(* Logix 5000 AddOnInstructionDefinition export EH_PicomagInsertion_DMI_IOL; software revision 38.00 *)

TYPE EH_CommAOI_Data :
STRUCT
   Device_Comm_Error : BOOL;
   CommSuccess : BOOL;
   CommFailed : BOOL;
   CommTimeOut : BOOL;
   StateDone : BOOL;
   NewState : BOOL;
   OldState : SINT;
   PortSize : SINT;
   DevicePort : SINT;
   MaxState : SINT;
   State : SINT;
   VendorID : INT;
   DeviceID : DINT;
   CyclicData : INT[16];
   AcyclicData : DINT[8];
   ReplayIndex : INT;
   AOI_Diagnostic : DINT;
   ConnectionStatus : DINT;
   OutputData : INT[16];
END_STRUCT
END_TYPE

ADD_ON_INSTRUCTION EH_PicomagInsertion_DMI_IOL   (* revision 1.0, vendor Endress+Hauser *)
// Picomag Insertion DMI Rev 1 IO-Link
VAR_IN_OUT
   DataToSend : INT[10]; {required}
   CommAOIBusy : DINT; {required}
   ActiveComPort : DINT; {required}
   DeviceAOISendRequest : DINT; {required}
   CommError : INT; {required}
   DeviceData : EH_CommAOI_Data; {required}
END_VAR
VAR_INPUT
   iSetSimulation : BOOL; {visible}
   iSimulation_OnOff : SINT; {access None, visible}
   iSimulationValue_FlowVelocity : REAL; {visible}
   iSimulationValue_Temperature : REAL; {visible}
   iSimulationValue_Conductivity : REAL; {visible}
   iSetTotalizerPresetValue : BOOL; {visible}
   iTotalizerPresetValue : REAL; {visible}
   iResetTotalizer : BOOL; {visible}
   iReadExtendedProcessData : BOOL; {access None, visible}
   iSetUnits : BOOL; {visible}
   iUnitConductivity : SINT; {visible}
   iUnitTotalizer : INT; {access None, visible}
   iUnitTemperature : SINT; {visible}
   iUnitFlowVelocity : INT; {visible}
   iUnitVolumeFlow : SINT; {visible}
END_VAR
VAR_OUTPUT
   qVendor_ID : DINT; {access Read Only, visible}
   qDevice_ID : DINT; {access Read Only, visible}
   qConductivity : REAL; {access None, visible}
   qVolumeTotalizer : REAL; {access None, visible}
   qTemperature : REAL; {visible}
   qFlowVelocity : REAL; {visible}
   qExtendedDeviceStatus : INT; {access Read Only, visible}
   qRelativeFlowRate : REAL; {access None, visible}
   qVolumeFlow : REAL; {access None, visible}
   qUnitConductivity : SINT; {access None, visible}
   qUnitTotalizer : INT; {access None, visible}
   qUnitTemperature : SINT; {access None, visible}
   qUnitFlowVelocity : INT; {access None, visible}
   qUnitVolumeFlow : SINT; {access None, visible}
   qAOI_Diagnostic : DINT; {access Read Only, visible}
END_VAR
VAR_IN_OUT
   qAOI_Diagnostic_String : STRING; {required}
END_VAR
VAR_OUTPUT
   qActual_Diagnostics_Code : DINT; {access Read Only, visible}
END_VAR
VAR_IN_OUT
   qActual_Diagnostics_String : STRING; {required}
END_VAR
VAR_OUTPUT
   qCommError : DINT; {access None}
   qCommunicationBusy : DINT; {access Read Only, visible}
   qDeviceConnectionError : BOOL; {access Read Only, visible}
END_VAR
VAR
   Temp_DINT : DINT; {access None}
   CMD_Index : INT; {access None}
   CMD_Subindex : INT; {access None}
   CMD_ByteLength : INT; {access None}
   oldCondStatus : INT; {access None}
   SetSimulation : SINT; {access None}
   SetTotalizerPresetValue : SINT; {access None}
   oldSetTotalizerPresetValue : SINT; {access None}
   oldSetSimulation : SINT; {access None}
   Trigger : BOOL; {access None}
   CMD_Rd : BOOL; {access None}
   CMD_Wr : BOOL; {access None}
   SimulationDINT : DINT; {access None}
   AOI_Prio : BOOL; {access None}
   StateMin : DINT; {access None}
   firstTimeDone : BOOL; {access None}
   CondStatusChanged : BOOL; {access None}
   Calc_Temperature : DINT; {access None}
   Calc_ExtendedDeviceStatus : DINT; {access None}
   CondStatusActive : BOOL; {access None}
   ActiveAOI : BOOL; {access None}
   TotActive : BOOL; {access None}
   Skip : BOOL; {access None}
   SetPulseSimulation : SINT; {access None}
   Calc_FlowVelocity : SINT; {access None}
   Calc_Totalizer : SINT; {access None}
   Calc_Conductivity : SINT; {access None}
   TotPresetChanged : BOOL; {access None}
   DeviceID : DINT; {access None}
   ResetTotalizerValue : SINT; {access None}
   oldResetTotalizerValue : SINT; {access None}
   SetUnits : SINT; {access None}
   oldSetUnits : SINT; {access None}
   SimChanged : BOOL; {access None}
   TRUE : BOOL := 1; {access None}
   FALSE : BOOL; {access None}
   SimActive : BOOL; {access None}
   temp_string1 : STRING; {access None}
   temp_string2 : STRING; {access None}
   tGradientConductivity : REAL; {access None}
   qConductivityTemp : REAL; {access None}
   qTemperatureTemp : REAL; {access None}
   qFlowVelocityTemp : REAL; {access None}
   tGradientFlowVelocity : REAL; {access None}
   qTotalizerTemp : REAL; {access None}
   qVolumeFlowTemp : REAL; {access None}
   qRelativeFlowRateTemp : REAL; {access None}
   ReadExtendedProcessData : SINT; {access None}
   oldReadExtendedProcessData : SINT; {access None}
   SetSimulation_OnOff : SINT; {access None}
   TotResetChanged : BOOL; {access None}
   UnitChanged : BOOL; {access None}
   UnitActive : BOOL; {access None}
   TotPresetActive : BOOL; {access None}
   TotResetActive : BOOL; {access None}
   ReadProcessDataChanged : BOOL; {access None}
   ReadProcessDataActive : BOOL; {access None}
   iSimulationValue_FlowVelocityTemp : REAL; {access None}
   SimulationValue_ConductivityTemp : REAL; {access None}
   qRelativeFlowRate_DINT : DINT; {access None}
   qVolumeFlow_DINT : DINT; {access None}
   iTotalizerPresetValueTemp : REAL; {access None}
   unit_check : BOOL; {access None}
   init_qUnits : BOOL; {access None}
   Underline_string : STRING; {access None}
END_VAR

ROUTINE Logic   (* structured text *)
// Picomag Communication via AL1323
   // =======================================================================
   // Endress+Hauser Digital Solutions
   // ©Copyright (2024) All Rights Reserved
   // =======================================================================
   // Name:                EH_PicomagInsertion_DMI_IOL
   // Version:             1.0
   // Datum:               11.2025
   // Library:             01.01.00
   // Engineering:         Studio5000 V38.00.00
   // Author:              EH
   // =======================================================================
   
   qAOI_Diagnostic := DeviceData.AOI_Diagnostic;
   qCommunicationBusy := CommAOIBusy;
   DeviceID := 9728001;
   StateMin := 0;
   DeviceData.MaxState := 98;
   temp_string1 := 'Error in step ';
   Underline_string := '----';
   
   if DeviceData.DevicePort = 0 or DeviceData.DeviceID <> DeviceID or DeviceData.ConnectionStatus <> 1 then
   
   	qVendor_ID := DeviceData.VendorID;
   	qDevice_ID := DeviceData.DeviceID;
   	qFlowVelocity := 0;
   	qTemperature := 0;
   	qFlowVelocity := 0;
   	qVolumeTotalizer := 0;
   	qRelativeFlowRate := 0;
   	qVolumeFlow := 0;
   	qConductivity := 0;
   	qUnitConductivity := 0;
   	qUnitTotalizer := 0;
   	qUnitTemperature := 0;
   	qUnitFlowVelocity := 0;
   	qUnitVolumeFlow := 0;
   	qExtendedDeviceStatus := 0;
   	qActual_Diagnostics_Code	:= 0;
   	DELETE(qActual_Diagnostics_String,1,1,qActual_Diagnostics_String);
   	oldCondStatus := 0;
   	CondStatusChanged := FALSE;
   	init_qUnits := FALSE;
   
   	if DeviceData.DevicePort = 0 then
   
   		qAOI_Diagnostic_String := 'Device port is zero';
   
   	elsif DeviceData.ConnectionStatus <> 1 then
   
   		qAOI_Diagnostic_String := 'No device connected';
   
   	elsif DeviceData.DeviceID <> DeviceID then
   
   		qAOI_Diagnostic_String := 'Wrong device ID';
   
   	end_if;
   
   else
   
   	if qActual_Diagnostics_Code = 0  then
   
   		CONCAT(Underline_string,Underline_string,qActual_Diagnostics_String);
   
   	end_if;
   
   	DELETE(qAOI_Diagnostic_String,1,1,qAOI_Diagnostic_String);
   	DeviceData.AOI_Diagnostic.1 := FALSE;
   	qDeviceConnectionError := FALSE;
   	DeviceData.AOI_Diagnostic.2  := FALSE;
   
   end_if;
   
   // Case device disconnected during communication to avoid blocking the communication
   if (DeviceData.AOI_Diagnostic.0 or qDeviceConnectionError or DeviceData.AOI_Diagnostic.2) and ActiveAOI and ActiveComPort = DeviceData.DevicePort and CommAOIBusy = 1 then
   
   	DeviceData.State := 0;
   	CommAOIBusy := 0;
   	DeviceAOISendRequest.[DeviceData.DevicePort] := 0;
   	ActiveComPort := 0;
   	ActiveAOI := 0;
   	DataToSend[0] := 0;
   	DataToSend[1] := 0;
   	DataToSend[2] := 0;
   	DataToSend[3] := 0;
   	DataToSend[4] := 0;
   	DataToSend[5] := 0;
   	DataToSend[6] := 0;
   	DataToSend[7] := 0;
   	DataToSend[8] := 0;
   	DataToSend[9] := 0;
   	DeviceData.StateDone := FALSE;
   	DeviceData.NewState := FALSE;
   	DeviceData.OldState := 0;
   	ActiveAOI := FALSE;
   
   end_if;
   
   if not DeviceData.AOI_Diagnostic.0
   	and not qDeviceConnectionError
   	and not DeviceData.AOI_Diagnostic.2
   	and DeviceData.DevicePort > 0 then
   
   	//*********************************
   	//Vendor ID
   	//*********************************
   
   		qVendor_ID := DeviceData.VendorID;
   
   	//*********************************
   	//Device ID
   	//*********************************
   
   		qDevice_ID := DeviceData.DeviceID;
   
   	//*********************************
   	// Picomag Insertion
   	//*********************************
   		Calc_Conductivity		    := 0;
   		Calc_Totalizer				:= 2;
   		Calc_Temperature			:= 4;
   		Calc_FlowVelocity			:= 6;
   		Calc_ExtendedDeviceStatus	:= 8;
   
   
   	//*********************************
   	//Process Data Conductivity
   	//*********************************
   
   		Temp_DINT	 := DeviceData.CyclicData[Calc_Conductivity+1];
   		Temp_DINT.8	 := DeviceData.CyclicData[Calc_Conductivity+1].8;
   		Temp_DINT.9  := DeviceData.CyclicData[Calc_Conductivity+1].9;
   		Temp_DINT.10 := DeviceData.CyclicData[Calc_Conductivity+1].10;
   		Temp_DINT.11 := DeviceData.CyclicData[Calc_Conductivity+1].11;
   		Temp_DINT.12 := DeviceData.CyclicData[Calc_Conductivity+1].12;
   		Temp_DINT.13 := DeviceData.CyclicData[Calc_Conductivity+1].13;
   		Temp_DINT.14 := DeviceData.CyclicData[Calc_Conductivity+1].14;
   		Temp_DINT.15 := DeviceData.CyclicData[Calc_Conductivity+1].15;
   		Temp_DINT.16 := DeviceData.CyclicData[Calc_Conductivity].0;
   		Temp_DINT.17 := DeviceData.CyclicData[Calc_Conductivity].1;
   		Temp_DINT.18 := DeviceData.CyclicData[Calc_Conductivity].2;
   		Temp_DINT.19 := DeviceData.CyclicData[Calc_Conductivity].3;
   		Temp_DINT.20 := DeviceData.CyclicData[Calc_Conductivity].4;
   		Temp_DINT.21 := DeviceData.CyclicData[Calc_Conductivity].5;
   		Temp_DINT.22 := DeviceData.CyclicData[Calc_Conductivity].6;
   		Temp_DINT.23 := DeviceData.CyclicData[Calc_Conductivity].7;
   		Temp_DINT.24 := DeviceData.CyclicData[Calc_Conductivity].8;
   		Temp_DINT.25 := DeviceData.CyclicData[Calc_Conductivity].9;
   		Temp_DINT.26 := DeviceData.CyclicData[Calc_Conductivity].10;
   		Temp_DINT.27 := DeviceData.CyclicData[Calc_Conductivity].11;
   		Temp_DINT.28 := DeviceData.CyclicData[Calc_Conductivity].12;
   		Temp_DINT.29 := DeviceData.CyclicData[Calc_Conductivity].13;
   		Temp_DINT.30 := DeviceData.CyclicData[Calc_Conductivity].14;
   		Temp_DINT.31 := DeviceData.CyclicData[Calc_Conductivity].15;
   
   		COP(Temp_DINT,qConductivityTemp,1);
   
   	//*********************************
   	// Process Data Volume Totalizer
   	//*********************************
   
   		Temp_DINT	 := DeviceData.CyclicData[Calc_Totalizer+1];
   		Temp_DINT.8  := DeviceData.CyclicData[Calc_Totalizer+1].8;
   		Temp_DINT.9  := DeviceData.CyclicData[Calc_Totalizer+1].9;
   		Temp_DINT.10 := DeviceData.CyclicData[Calc_Totalizer+1].10;
   		Temp_DINT.11 := DeviceData.CyclicData[Calc_Totalizer+1].11;
   		Temp_DINT.12 := DeviceData.CyclicData[Calc_Totalizer+1].12;
   		Temp_DINT.13 := DeviceData.CyclicData[Calc_Totalizer+1].13;
   		Temp_DINT.14 := DeviceData.CyclicData[Calc_Totalizer+1].14;
   		Temp_DINT.15 := DeviceData.CyclicData[Calc_Totalizer+1].15;
   		Temp_DINT.16 := DeviceData.CyclicData[Calc_Totalizer].0;
   		Temp_DINT.17 := DeviceData.CyclicData[Calc_Totalizer].1;
   		Temp_DINT.18 := DeviceData.CyclicData[Calc_Totalizer].2;
   		Temp_DINT.19 := DeviceData.CyclicData[Calc_Totalizer].3;
   		Temp_DINT.20 := DeviceData.CyclicData[Calc_Totalizer].4;
   		Temp_DINT.21 := DeviceData.CyclicData[Calc_Totalizer].5;
   		Temp_DINT.22 := DeviceData.CyclicData[Calc_Totalizer].6;
   		Temp_DINT.23 := DeviceData.CyclicData[Calc_Totalizer].7;
   		Temp_DINT.24 := DeviceData.CyclicData[Calc_Totalizer].8;
   		Temp_DINT.25 := DeviceData.CyclicData[Calc_Totalizer].9;
   		Temp_DINT.26 := DeviceData.CyclicData[Calc_Totalizer].10;
   		Temp_DINT.27 := DeviceData.CyclicData[Calc_Totalizer].11;
   		Temp_DINT.28 := DeviceData.CyclicData[Calc_Totalizer].12;
   		Temp_DINT.29 := DeviceData.CyclicData[Calc_Totalizer].13;
   		Temp_DINT.30 := DeviceData.CyclicData[Calc_Totalizer].14;
   		Temp_DINT.31 := DeviceData.CyclicData[Calc_Totalizer].15;
   
   		COP(Temp_DINT,qTotalizerTemp,1);
   
   	//*********************************
   	// Process Data Temperature
   	//*********************************
   
   		Temp_DINT	 := DeviceData.CyclicData[Calc_Temperature+1];
   		Temp_DINT.8	 := DeviceData.CyclicData[Calc_Temperature+1].8;
   		Temp_DINT.9	 := DeviceData.CyclicData[Calc_Temperature+1].9;
   		Temp_DINT.10 := DeviceData.CyclicData[Calc_Temperature+1].10;
   		Temp_DINT.11 := DeviceData.CyclicData[Calc_Temperature+1].11;
   		Temp_DINT.12 := DeviceData.CyclicData[Calc_Temperature+1].12;
   		Temp_DINT.13 := DeviceData.CyclicData[Calc_Temperature+1].13;
   		Temp_DINT.14 := DeviceData.CyclicData[Calc_Temperature+1].14;
   		Temp_DINT.15 := DeviceData.CyclicData[Calc_Temperature+1].15;
   		Temp_DINT.16 := DeviceData.CyclicData[Calc_Temperature].0;
   		Temp_DINT.17 := DeviceData.CyclicData[Calc_Temperature].1;
   		Temp_DINT.18 := DeviceData.CyclicData[Calc_Temperature].2;
   		Temp_DINT.19 := DeviceData.CyclicData[Calc_Temperature].3;
   		Temp_DINT.20 := DeviceData.CyclicData[Calc_Temperature].4;
   		Temp_DINT.21 := DeviceData.CyclicData[Calc_Temperature].5;
   		Temp_DINT.22 := DeviceData.CyclicData[Calc_Temperature].6;
   		Temp_DINT.23 := DeviceData.CyclicData[Calc_Temperature].7;
   		Temp_DINT.24 := DeviceData.CyclicData[Calc_Temperature].8;
   		Temp_DINT.25 := DeviceData.CyclicData[Calc_Temperature].9;
   		Temp_DINT.26 := DeviceData.CyclicData[Calc_Temperature].10;
   		Temp_DINT.27 := DeviceData.CyclicData[Calc_Temperature].11;
   		Temp_DINT.28 := DeviceData.CyclicData[Calc_Temperature].12;
   		Temp_DINT.29 := DeviceData.CyclicData[Calc_Temperature].13;
   		Temp_DINT.30 := DeviceData.CyclicData[Calc_Temperature].14;
   		Temp_DINT.31 := DeviceData.CyclicData[Calc_Temperature].15;
   
   		COP(Temp_DINT,qTemperatureTemp,1);
   
   	//*********************************
   	// Process Data Flow Velocity
   	//*********************************
   
   		Temp_DINT	 := DeviceData.CyclicData[Calc_FlowVelocity+1];
   		Temp_DINT.8  := DeviceData.CyclicData[Calc_FlowVelocity+1].8;
   		Temp_DINT.9  := DeviceData.CyclicData[Calc_FlowVelocity+1].9;
   		Temp_DINT.10 := DeviceData.CyclicData[Calc_FlowVelocity+1].10;
   		Temp_DINT.11 := DeviceData.CyclicData[Calc_FlowVelocity+1].11;
   		Temp_DINT.12 := DeviceData.CyclicData[Calc_FlowVelocity+1].12;
   		Temp_DINT.13 := DeviceData.CyclicData[Calc_FlowVelocity+1].13;
   		Temp_DINT.14 := DeviceData.CyclicData[Calc_FlowVelocity+1].14;
   		Temp_DINT.15 := DeviceData.CyclicData[Calc_FlowVelocity+1].15;
   		Temp_DINT.16 := DeviceData.CyclicData[Calc_FlowVelocity].0;
   		Temp_DINT.17 := DeviceData.CyclicData[Calc_FlowVelocity].1;
   		Temp_DINT.18 := DeviceData.CyclicData[Calc_FlowVelocity].2;
   		Temp_DINT.19 := DeviceData.CyclicData[Calc_FlowVelocity].3;
   		Temp_DINT.20 := DeviceData.CyclicData[Calc_FlowVelocity].4;
   		Temp_DINT.21 := DeviceData.CyclicData[Calc_FlowVelocity].5;
   		Temp_DINT.22 := DeviceData.CyclicData[Calc_FlowVelocity].6;
   		Temp_DINT.23 := DeviceData.CyclicData[Calc_FlowVelocity].7;
   		Temp_DINT.24 := DeviceData.CyclicData[Calc_FlowVelocity].8;
   		Temp_DINT.25 := DeviceData.CyclicData[Calc_FlowVelocity].9;
   		Temp_DINT.26 := DeviceData.CyclicData[Calc_FlowVelocity].10;
   		Temp_DINT.27 := DeviceData.CyclicData[Calc_FlowVelocity].11;
   		Temp_DINT.28 := DeviceData.CyclicData[Calc_FlowVelocity].12;
   		Temp_DINT.29 := DeviceData.CyclicData[Calc_FlowVelocity].13;
   		Temp_DINT.30 := DeviceData.CyclicData[Calc_FlowVelocity].14;
   		Temp_DINT.31 := DeviceData.CyclicData[Calc_FlowVelocity].15;
   
   		COP(Temp_DINT,qFlowVelocityTemp,1);
   
   	//*********************************
   	// Units handling
   	//*********************************
   		case qUnitConductivity of
   
   			//*********************************
   			3: // S/m
   			//*********************************
   				tGradientConductivity := 0.0001;
   
   			//*********************************
   			6: // mS/cm
   			//*********************************
   				tGradientConductivity := 0.001;
   
   			//*********************************
   			8: // uS/cm
   			//*********************************
   				tGradientConductivity := 1.0;
   
   			else // Base unit
   				tGradientConductivity := 1.0;
   
   		end_case;
   
   		qConductivity := qConductivityTemp * tGradientConductivity;
   
   		case qUnitTotalizer of
   
   			//*********************************
   			2: // m³
   			//*********************************
   				qVolumeTotalizer := qTotalizerTemp * 0.001;
   
   			//*********************************
   			4: // l
   			//*********************************
   				qVolumeTotalizer := qTotalizerTemp;
   
   			//*********************************
   			10: // fl oz (us)
   			//*********************************
   				qVolumeTotalizer := qTotalizerTemp * 33.814;
   
   			//*********************************
   			11: // gal(us)
   			//*********************************
   				qVolumeTotalizer := qTotalizerTemp * 0.264172;
   
   			//*********************************
   			22: // kgal (us)
   			//*********************************
   				qVolumeTotalizer := qTotalizerTemp * 0.000264;
   
   			//*********************************
   			150: // kl
   			//*********************************
   				qVolumeTotalizer := qTotalizerTemp * 0.001;
   
   			else // Base unit
   				qVolumeTotalizer := qTotalizerTemp;
   
   		end_case;
   
   		case qUnitTemperature of
   
   			//*********************************
   			32: // °C
   			//*********************************
   				qTemperature := qTemperatureTemp;
   
   			//*********************************
   			33: // °F
   			//*********************************
   				qTemperature := qTemperatureTemp * 9.0 / 5.0 + 32;
   
   			else // °C
   				qTemperature := qTemperatureTemp;
   
   		end_case;
   
   	    case qUnitFlowVelocity of
   	        21: // m/s
   	            tGradientFlowVelocity := 1.0;
   	        22: // ft/s
   	            tGradientFlowVelocity := 3.28084;
   	        50: // ft/h
   	            tGradientFlowVelocity := 11811.02362;
   	        114: // in/s
   	            tGradientFlowVelocity := 39.3701;
   	        115: // in/min
   	            tGradientFlowVelocity := 2362.2;
   	        116: // ft/min
   	            tGradientFlowVelocity := 196.85;
   	        120: // m/h
   	            tGradientFlowVelocity := 3600;
   	        240: // in/h
   	            tGradientFlowVelocity := 141732.2835;
   	        else // m/s
   	            tGradientFlowVelocity := 1.0;
   	    end_case;
   
   	    qFlowVelocity := qFlowVelocityTemp * tGradientFlowVelocity;
   
       	case qUnitVolumeFlow of
   	        16: // gal/min (us)
   	            qVolumeFlow := qVolumeFlowTemp * 18.8503;
   	        17: // l/min
   	            qVolumeFlow := qVolumeFlowTemp * 60;
   	        18: // l/h
   	            qVolumeFlow := qVolumeFlowTemp * 3600;
   	        19: // m³/h
   	            qVolumeFlow := qVolumeFlowTemp * 3.6;
   	        24: // l/s
   	            qVolumeFlow := qVolumeFlowTemp;
   	        41: // fl oz/min
   	            qVolumeFlow := qVolumeFlowTemp * 2028.84;
   	        ELSE // l/s
   	            qVolumeFlow := qVolumeFlowTemp;
   	    end_case;
   
   
   	//*********************************
   	// Extended device Status
   	//*********************************
   
   		qExtendedDeviceStatus.0 := DeviceData.CyclicData[Calc_ExtendedDeviceStatus].8;
   		qExtendedDeviceStatus.1 := DeviceData.CyclicData[Calc_ExtendedDeviceStatus].9;
   		qExtendedDeviceStatus.2 := DeviceData.CyclicData[Calc_ExtendedDeviceStatus].10;
   		qExtendedDeviceStatus.3 := DeviceData.CyclicData[Calc_ExtendedDeviceStatus].11;
   		qExtendedDeviceStatus.4 := DeviceData.CyclicData[Calc_ExtendedDeviceStatus].12;
   		qExtendedDeviceStatus.5 := DeviceData.CyclicData[Calc_ExtendedDeviceStatus].13;
   		qExtendedDeviceStatus.6 := DeviceData.CyclicData[Calc_ExtendedDeviceStatus].14;
   		qExtendedDeviceStatus.7 := DeviceData.CyclicData[Calc_ExtendedDeviceStatus].15;
   
   
   	//*********************************
   	// Checking for Changed Status
   	//*********************************
   
   		SetSimulation.0 := iSetSimulation;
   		SetTotalizerPresetValue.0 := iSetTotalizerPresetValue;
   		ResetTotalizerValue.0 := iResetTotalizer;
   		SetUnits.0 := iSetUnits;
   		ReadExtendedProcessData.0 := iReadExtendedProcessData;
   
   		// Condensed status
   		if oldCondStatus <> qExtendedDeviceStatus and not CondStatusChanged then
   
   			CondStatusChanged := TRUE;
   			oldCondStatus := qExtendedDeviceStatus;
   
   		end_if;
   
   		// Set simulation
   		if oldSetSimulation <> SetSimulation and not SimChanged then
   
   			if oldSetSimulation <> SetSimulation then
   
   				SimChanged := TRUE;
   
   			end_if;
   
   			oldSetSimulation := SetSimulation;
   
   		end_if;
   
   		// Set totalizer preset value
   		if oldSetTotalizerPresetValue <> SetTotalizerPresetValue and not TotPresetChanged then
   
   			if oldSetTotalizerPresetValue < SetTotalizerPresetValue then
   
   				TotPresetChanged := TRUE;
   
   			end_if;
   
   			oldSetTotalizerPresetValue := SetTotalizerPresetValue;
   
   		end_if;
   
   		// Reset totalizer value
   		if oldResetTotalizerValue <> ResetTotalizerValue and not TotResetChanged then
   
   			if oldResetTotalizerValue < ResetTotalizerValue then
   
   				TotResetChanged := TRUE;
   
   			end_if;
   
   			oldResetTotalizerValue := ResetTotalizerValue;
   
   		end_if;
   
   		// Set units
   		if oldSetUnits <> SetUnits and not UnitChanged then
   
   			if oldSetUnits < SetUnits then
   
   				UnitChanged := TRUE;
   
   			end_if;
   
   			oldSetUnits := SetUnits;
   
   		end_if;
   
   		// Read extended process data
   		if oldReadExtendedProcessData <> ReadExtendedProcessData and not ReadProcessDataChanged then
   
   			if oldReadExtendedProcessData < ReadExtendedProcessData then
   
   				ReadProcessDataChanged := TRUE;
   
   			end_if;
   
   			oldReadExtendedProcessData := ReadExtendedProcessData;
   
   		end_if;
   
   		if CondStatusChanged
   		and not ActiveAOI
   		and not CondStatusActive
   		and not Skip then
   
   			DeviceAOISendRequest.[DeviceData.DevicePort] := TRUE;
   			CondStatusActive := TRUE;
   			Skip := TRUE;
   
   		elsif SimChanged
   			and not ActiveAOI
   			and not SimActive
   			and not Skip then
   
   			DeviceAOISendRequest.[DeviceData.DevicePort] := TRUE;
   			SimActive := TRUE;
   			Skip := TRUE;
   
   		elsif ReadProcessDataChanged
   			and not ActiveAOI
   			and not ReadProcessDataActive
   			and not Skip then
   
   			DeviceAOISendRequest.[DeviceData.DevicePort] := TRUE;
   			ReadProcessDataActive := TRUE;
   			Skip := TRUE;
   
   		elsif TotPresetChanged
   			and not ActiveAOI
   			and not TotPresetActive
   			and not Skip then
   
   			DeviceAOISendRequest.[DeviceData.DevicePort] := TRUE;
   			TotPresetActive := TRUE;
   			Skip := TRUE;
   
   		elsif TotResetChanged
   			and not ActiveAOI
   			and not TotResetActive
   			and not Skip then
   
   			DeviceAOISendRequest.[DeviceData.DevicePort] := TRUE;
   			TotResetActive := TRUE;
   			Skip := TRUE;
   
   		elsif UnitChanged
   			and not ActiveAOI
   			and not UnitActive
   			and not Skip then
   
   			DeviceAOISendRequest.[DeviceData.DevicePort] := TRUE;
   			UnitActive := TRUE;
   			Skip := TRUE;
   
   
   		end_if;
   
   		if ActiveComPort = DeviceData.DevicePort then
   
   			AOI_Prio :=TRUE;
   
   		else
   
   			AOI_Prio := FALSE;
   
   		end_if;
   
   		if (CondStatusActive or SimActive or TotPresetActive or TotResetActive or UnitActive or ReadProcessDataActive) and CommAOIBusy = 1  and DeviceData.State = 0 and AOI_Prio and not ActiveAOI then
   
   			ActiveAOI := TRUE;
   			Skip := FALSE;
   
   		end_if;
   
   		qCommunicationBusy := CommAOIBusy;
   		qAOI_Diagnostic :=DeviceData.AOI_Diagnostic;
   
   	//*********************************
   	// States for Execution
   	//*********************************
   
   	if ActiveAOI or DeviceData.State = DeviceData.MaxState then
   
   	case DeviceData.State of
   
   		//*********************************
   		0: // Idle
   		//*********************************
   
   			// Initializing
   			Trigger := FALSE;
   			CMD_Index := 0;
   			CMD_Subindex := 0;
   			CMD_Wr := FALSE;
   			CMD_Rd := FALSE;
   		    CMD_ByteLength := 0;
   
   			if DeviceData.DevicePort = ActiveComPort then
   
   					DeviceData.CommSuccess := FALSE;
   					DeviceData.CommTimeOut := FALSE;
   					DeviceData.NewState := TRUE;
   					DeviceData.StateDone := FALSE;
   
   			end_if;
   
   			// Wait for trigger
   			// Set Simulation
   			if SimActive then
   
   				DeviceData.AOI_Diagnostic := 0;
   				DeviceData.State := 1;
   
   			// Read extended process data
   			elsif ReadProcessDataActive then
   
   				DeviceData.AOI_Diagnostic := 0;
   				DeviceData.State := 10;
   
   			// Set totalizer preset value
   			elsif TotPresetActive then
   
   				DeviceData.AOI_Diagnostic := 0;
   				DeviceData.State := 20;
   
   			 // Reset totalizer value
   			elsif TotResetActive then
   
   				DeviceData.AOI_Diagnostic := 0;
   				DeviceData.State := 21;
   
   			 // Set units
   			elsif UnitActive then
   
   				DeviceData.AOI_Diagnostic := 0;
   				DeviceData.State := 30;
   
   			// Update diagnostics
   			elsif CondStatusChanged then
   
   				if not init_qUnits then
   
   					DeviceData.State := 35;
   
   				else
   
   					DeviceData.State := 90;
   
   				end_if;
   
   			end_if;
   
   		//*********************************************
   		1: // Set Simulation
   		//*********************************************
   			CMD_Index := 2066;
   			CMD_Subindex := 0;
   			CMD_Wr := TRUE;								// Only Read or Write can be active = 1
   			CMD_Rd := FALSE;
   			CMD_ByteLength := 2;
   			DataToSend[6]:= 0;
   			DataToSend[7]:= 0;
   
   			if iSimulation_OnOff = 0 then
   
   				DataToSend[6] := 0;
   				DataToSend[7] := 0;
   
   			else
   
   				DataToSend[6].8 := TRUE;
   				DataToSend[6].9 := SetSimulation_OnOff.1;
   				DataToSend[6].10 := SetSimulation_OnOff.2;
   				DataToSend[6].11 := SetSimulation_OnOff.3;
   				DataToSend[6].12 := SetSimulation_OnOff.4;
   				DataToSend[6].13 := SetSimulation_OnOff.5;
   				DataToSend[6].14 := SetSimulation_OnOff.6;
   				DataToSend[6].15 := SetSimulation_OnOff.7;
   
   			end_if;
   
   			Trigger := TRUE;
   
   			if DeviceData.NewState then
   
   				DeviceData.StateDone := TRUE;
   
   			end_if;
   
   			if  DeviceData.CommSuccess and DeviceData.ReplayIndex = CMD_Index then
   
   				Trigger := FALSE;
   				DeviceData.OldState := DeviceData.State;
   				DeviceData.State := DeviceData.State + 1;
   				DeviceData.CommSuccess := FALSE;
   				DeviceData.AcyclicData[0] := 0;
   				DeviceData.NewState := TRUE;
   
   			elsif DeviceData.CommTimeOut then
   
   				Temp_DINT := DeviceData.State;
   				DTOS(Temp_DINT, temp_string2);
   				CONCAT(temp_string1, temp_string2, qAOI_Diagnostic_String);
   
   				DeviceData.OldState := DeviceData.State;
   				DeviceData.State := DeviceData.MaxState;
   				DeviceData.CommTimeOut := FALSE;
   				DeviceData.AcyclicData[0] := 0;
   				DeviceData.NewState := TRUE;
   
   			end_if;
   
   		//*********************************************
   		2: // Set simulation value - flow velocity
   		//*********************************************
   			CMD_Index := 8292;
   			CMD_Subindex := 0;
   			CMD_Wr := TRUE;
   			CMD_Rd := FALSE;
   			CMD_ByteLength := 4;
   			DataToSend[6]:= 0;
   			DataToSend[7]:= 0;
   
   			// Convert simulation value in DINT
   			iSimulationValue_FlowVelocityTemp := iSimulationValue_FlowVelocity / tGradientFlowVelocity;
   			COP(iSimulationValue_FlowVelocityTemp,SimulationDINT,1); // Copy the Bits from the Real in a DINT
   
   			DataToSend[6].0 :=  SimulationDINT.24;
   			DataToSend[6].1 :=  SimulationDINT.25;
   			DataToSend[6].2 :=  SimulationDINT.26;
   			DataToSend[6].3 :=  SimulationDINT.27;
   			DataToSend[6].4 :=  SimulationDINT.28;
   			DataToSend[6].5 :=  SimulationDINT.29;
   			DataToSend[6].6 :=  SimulationDINT.30;
   			DataToSend[6].7 :=  SimulationDINT.31;
   			DataToSend[6].8 :=  SimulationDINT.16;
   			DataToSend[6].9 :=  SimulationDINT.17;
   			DataToSend[6].10 := SimulationDINT.18;
   			DataToSend[6].11 := SimulationDINT.19;
   			DataToSend[6].12 := SimulationDINT.20;
   			DataToSend[6].13 := SimulationDINT.21;
   			DataToSend[6].14 := SimulationDINT.22;
   			DataToSend[6].15 := SimulationDINT.23;
   			DataToSend[7].0  := SimulationDINT.8;
   			DataToSend[7].1  := SimulationDINT.9;
   			DataToSend[7].2  := SimulationDINT.10;
   			DataToSend[7].3  := SimulationDINT.11;
   			DataToSend[7].4  := SimulationDINT.12;
   			DataToSend[7].5  := SimulationDINT.13;
   			DataToSend[7].6  := SimulationDINT.14;
   			DataToSend[7].7  := SimulationDINT.15;
   			DataToSend[7].8  := SimulationDINT.0;
   			DataToSend[7].9  := SimulationDINT.1;
   			DataToSend[7].10 := SimulationDINT.2;
   			DataToSend[7].11 := SimulationDINT.3;
   			DataToSend[7].12 := SimulationDINT.4;
   			DataToSend[7].13 := SimulationDINT.5;
   			DataToSend[7].14 := SimulationDINT.6;
   			DataToSend[7].15 := SimulationDINT.7;
   
   			Trigger := TRUE;
   
   			if DeviceData.NewState then
   
   				DeviceData.StateDone := TRUE;
   
   			end_if;
   
   			if  DeviceData.CommSuccess and DeviceData.ReplayIndex = CMD_Index then
   
   				Trigger := FALSE;
   				DeviceData.OldState := DeviceData.State;
   				DeviceData.State := DeviceData.State + 1;
   				DeviceData.CommSuccess := FALSE;
   				DeviceData.AcyclicData[0] := 0;
   				DeviceData.NewState := TRUE;
   
   			elsif DeviceData.CommTimeOut then
   
   				Temp_DINT := DeviceData.State;
   				DTOS(Temp_DINT, temp_string2);
   				CONCAT(temp_string1, temp_string2, qAOI_Diagnostic_String);
   
   				DeviceData.OldState := DeviceData.State;
   				DeviceData.State := DeviceData.MaxState;
   				DeviceData.CommTimeOut := FALSE;
   				DeviceData.AcyclicData[0] := 0;
   				DeviceData.NewState := TRUE;
   
   			end_if;
   
   
   		//*********************************************
   		3: // Set simulation value - temperature
   		//*********************************************
   			CMD_Index := 8279;
   			CMD_Subindex := 0;
   			CMD_Wr := TRUE;
   			CMD_Rd := FALSE;
   			CMD_ByteLength := 4;
   			DataToSend[6]:= 0;
   			DataToSend[7]:= 0;
   
   			case qUnitTemperature of
   
   				//*********************************
   				32: // °C
   				//*********************************
   					iSimulationValue_Temperature := iSimulationValue_Temperature;
   
   				//*********************************
   				33: // °F
   				//*********************************
   					iSimulationValue_Temperature := (iSimulationValue_Temperature -32)*5/9;
   
   				else // °C
   					iSimulationValue_Temperature := iSimulationValue_Temperature;
   
   			end_case;
   
   			// Convert simulation value in DINT
   			COP(iSimulationValue_Temperature,SimulationDINT,1);
   
   			DataToSend[6].0 :=  SimulationDINT.24;
   			DataToSend[6].1 :=  SimulationDINT.25;
   			DataToSend[6].2 :=  SimulationDINT.26;
   			DataToSend[6].3 :=  SimulationDINT.27;
   			DataToSend[6].4 :=  SimulationDINT.28;
   			DataToSend[6].5 :=  SimulationDINT.29;
   			DataToSend[6].6 :=  SimulationDINT.30;
   			DataToSend[6].7 :=  SimulationDINT.31;
   			DataToSend[6].8 :=  SimulationDINT.16;
   			DataToSend[6].9 :=  SimulationDINT.17;
   			DataToSend[6].10 := SimulationDINT.18;
   			DataToSend[6].11 := SimulationDINT.19;
   			DataToSend[6].12 := SimulationDINT.20;
   			DataToSend[6].13 := SimulationDINT.21;
   			DataToSend[6].14 := SimulationDINT.22;
   			DataToSend[6].15 := SimulationDINT.23;
   			DataToSend[7].0  := SimulationDINT.8;
   			DataToSend[7].1  := SimulationDINT.9;
   			DataToSend[7].2  := SimulationDINT.10;
   			DataToSend[7].3  := SimulationDINT.11;
   			DataToSend[7].4  := SimulationDINT.12;
   			DataToSend[7].5  := SimulationDINT.13;
   			DataToSend[7].6  := SimulationDINT.14;
   			DataToSend[7].7  := SimulationDINT.15;
   			DataToSend[7].8  := SimulationDINT.0;
   			DataToSend[7].9  := SimulationDINT.1;
   			DataToSend[7].10 := SimulationDINT.2;
   			DataToSend[7].11 := SimulationDINT.3;
   			DataToSend[7].12 := SimulationDINT.4;
   			DataToSend[7].13 := SimulationDINT.5;
   			DataToSend[7].14 := SimulationDINT.6;
   			DataToSend[7].15 := SimulationDINT.7;
   
   			Trigger := TRUE;
   
   			if DeviceData.NewState then
   
   				DeviceData.StateDone := TRUE;
   
   			end_if;
   
   			if  DeviceData.CommSuccess and DeviceData.ReplayIndex = CMD_Index then
   
   				Trigger := FALSE;
   				DeviceData.OldState := DeviceData.State;
   				DeviceData.State := DeviceData.State + 1;
   				DeviceData.CommSuccess := FALSE;
   				DeviceData.AcyclicData[0] := 0;
   				DeviceData.NewState := TRUE;
   
   			elsif DeviceData.CommTimeOut then
   
   				Temp_DINT := DeviceData.State;
   				DTOS(Temp_DINT, temp_string2);
   				CONCAT(temp_string1, temp_string2, qAOI_Diagnostic_String);
   
   				DeviceData.OldState := DeviceData.State;
   				DeviceData.State := DeviceData.MaxState;
   				DeviceData.CommTimeOut := FALSE;
   				DeviceData.AcyclicData[0] := 0;
   				DeviceData.NewState := TRUE;
   
   			end_if;
   
   
   		//*********************************************
   		4: // Set simulation value - conductivity
   		//*********************************************
   			CMD_Index := 8278;
   			CMD_Subindex := 0;
   			CMD_Wr := TRUE;
   			CMD_Rd := FALSE;
   			CMD_ByteLength := 4;
   			DataToSend[6]:= 0;
   			DataToSend[7]:= 0;
   
   			case qUnitConductivity of
   
   				//*********************************
   				3: // S/m
   				//*********************************
   					SimulationValue_ConductivityTemp := iSimulationValue_Conductivity;
   
   				//*********************************
   				6: // mS/cm
   				//*********************************
   					SimulationValue_ConductivityTemp := iSimulationValue_Conductivity * 0.1;
   
   				//*********************************
   				8: // uS/cm
   				//*********************************
   					SimulationValue_ConductivityTemp := iSimulationValue_Conductivity * 0.0001;
   
   				else // Base unit
   					SimulationValue_ConductivityTemp := iSimulationValue_Conductivity;
   
   			end_case;
   
   			// Convert simulation value in DINT
   			COP(SimulationValue_ConductivityTemp,SimulationDINT,1);
   
   			DataToSend[6].0 :=  SimulationDINT.24;
   			DataToSend[6].1 :=  SimulationDINT.25;
   			DataToSend[6].2 :=  SimulationDINT.26;
   			DataToSend[6].3 :=  SimulationDINT.27;
   			DataToSend[6].4 :=  SimulationDINT.28;
   			DataToSend[6].5 :=  SimulationDINT.29;
   			DataToSend[6].6 :=  SimulationDINT.30;
   			DataToSend[6].7 :=  SimulationDINT.31;
   			DataToSend[6].8 :=  SimulationDINT.16;
   			DataToSend[6].9 :=  SimulationDINT.17;
   			DataToSend[6].10 := SimulationDINT.18;
   			DataToSend[6].11 := SimulationDINT.19;
   			DataToSend[6].12 := SimulationDINT.20;
   			DataToSend[6].13 := SimulationDINT.21;
   			DataToSend[6].14 := SimulationDINT.22;
   			DataToSend[6].15 := SimulationDINT.23;
   			DataToSend[7].0  := SimulationDINT.8;
   			DataToSend[7].1  := SimulationDINT.9;
   			DataToSend[7].2  := SimulationDINT.10;
   			DataToSend[7].3  := SimulationDINT.11;
   			DataToSend[7].4  := SimulationDINT.12;
   			DataToSend[7].5  := SimulationDINT.13;
   			DataToSend[7].6  := SimulationDINT.14;
   			DataToSend[7].7  := SimulationDINT.15;
   			DataToSend[7].8  := SimulationDINT.0;
   			DataToSend[7].9  := SimulationDINT.1;
   			DataToSend[7].10 := SimulationDINT.2;
   			DataToSend[7].11 := SimulationDINT.3;
   			DataToSend[7].12 := SimulationDINT.4;
   			DataToSend[7].13 := SimulationDINT.5;
   			DataToSend[7].14 := SimulationDINT.6;
   			DataToSend[7].15 := SimulationDINT.7;
   
   			Trigger := TRUE;
   
   			if DeviceData.NewState then
   
   				DeviceData.StateDone := TRUE;
   
   			end_if;
   
   			if  DeviceData.CommSuccess and DeviceData.ReplayIndex = CMD_Index then
   
   				Trigger := FALSE;
   				DeviceData.OldState := DeviceData.State;
   				DeviceData.State := DeviceData.MaxState;
   				DeviceData.CommSuccess := FALSE;
   				DeviceData.AcyclicData[0] := 0;
   				DeviceData.NewState := TRUE;
   
   			elsif DeviceData.CommTimeOut then
   
   				Temp_DINT := DeviceData.State;
   				DTOS(Temp_DINT, temp_string2);
   				CONCAT(temp_string1, temp_string2, qAOI_Diagnostic_String);
   
   				DeviceData.OldState := DeviceData.State;
   				DeviceData.State := DeviceData.MaxState;
   				DeviceData.CommTimeOut := FALSE;
   				DeviceData.AcyclicData[0] := 0;
   				DeviceData.NewState := TRUE;
   
   			end_if;
   
   
   		//*********************************************
   		10: // Read relative flow rate
   		//*********************************************
   			CMD_Index := 8289;
   			CMD_Subindex := 0;
   			CMD_Wr := FALSE;
   			CMD_Rd := TRUE;
   			CMD_ByteLength := 4;
   			DataToSend[6]:= 0;
   			DataToSend[7]:= 0;
   
   			Trigger := TRUE;
   
   			if DeviceData.NewState then
   
   				DeviceData.StateDone := TRUE;
   
   			end_if;
   
   			if  DeviceData.CommSuccess and DeviceData.ReplayIndex = CMD_Index then
   
   				// Convert DINT to REAL
   				qRelativeFlowRate_DINT := DeviceData.AcyclicData[0];
   	 			COP(qRelativeFlowRate_DINT, qRelativeFlowRate,1);
   
   				Trigger := FALSE;
   				DeviceData.OldState := DeviceData.State;
   				DeviceData.State := DeviceData.State + 1;
   				DeviceData.CommSuccess := FALSE;
   				DeviceData.AcyclicData[0] := 0;
   				DeviceData.NewState := TRUE;
   
   			elsif DeviceData.CommTimeOut then
   
   				Temp_DINT := DeviceData.State;
   				DTOS(Temp_DINT, temp_string2);
   				CONCAT(temp_string1, temp_string2, qAOI_Diagnostic_String);
   
   				DeviceData.OldState := DeviceData.State;
   				DeviceData.State := DeviceData.MaxState;
   				DeviceData.CommTimeOut := FALSE;
   				DeviceData.AcyclicData[0] := 0;
   				DeviceData.NewState := TRUE;
   
   			end_if;
   
   		//***************************************
   		11: // Read volume flow
   		//***************************************
   			CMD_Index := 2068;
   			CMD_Subindex := 0;
   			CMD_Wr := FALSE;
   			CMD_Rd := TRUE;
   			CMD_ByteLength := 4;
   			DataToSend[6]:= 0;
   			DataToSend[7]:= 0;
   
   			Trigger := TRUE;
   
   			if DeviceData.NewState then
   
   				DeviceData.StateDone := TRUE;
   
   			end_if;
   
   			if  DeviceData.CommSuccess and DeviceData.ReplayIndex = CMD_Index then
   
   				// Convert DINT to REAL
   				qVolumeFlow_DINT := DeviceData.AcyclicData[0];
   	 			COP(qVolumeFlow_DINT, qVolumeFlowTemp,1);
   
   				Trigger := FALSE;
   				DeviceData.OldState := DeviceData.State;
   				DeviceData.State := DeviceData.MaxState;
   				DeviceData.CommSuccess := FALSE;
   				DeviceData.AcyclicData[0] := 0;
   				DeviceData.NewState := TRUE;
   
   			elsif DeviceData.CommTimeOut then
   
   				Temp_DINT := DeviceData.State;
   				DTOS(Temp_DINT, temp_string2);
   				CONCAT(temp_string1, temp_string2, qAOI_Diagnostic_String);
   
   				DeviceData.OldState := DeviceData.State;
   				DeviceData.State := DeviceData.MaxState;
   				DeviceData.CommTimeOut := FALSE;
   				DeviceData.AcyclicData[0] := 0;
   				DeviceData.NewState := TRUE;
   
   			end_if;
   
   		//*********************************
   		20: // Set totalizer preset value
   		//*********************************
   			CMD_Index := 8280;
   			CMD_Subindex := 0;
   			CMD_Wr := TRUE;
   			CMD_Rd := FALSE;
   			CMD_ByteLength := 4;
   			DataToSend[6]:= 0;
   			DataToSend[7]:= 0;
   
   			case qUnitTotalizer of
   
   				//*********************************
   				2: // m³
   				//*********************************
   					iTotalizerPresetValueTemp := iTotalizerPresetValue;
   
   				//*********************************
   				4: // l
   				//*********************************
   					iTotalizerPresetValueTemp := iTotalizerPresetValue/1000.0;
   
   				//*********************************
   				10: // fl oz (us)
   				//*********************************
   					iTotalizerPresetValueTemp := (iTotalizerPresetValue/33.814)/1000.0;
   
   				//*********************************
   				11: // gal(us)
   				//*********************************
   					iTotalizerPresetValueTemp := (iTotalizerPresetValue/0.264172)/1000.0;
   
   
   				//*********************************
   				22: // kgal (us)
   				//*********************************
   					iTotalizerPresetValueTemp := (iTotalizerPresetValue/0.000264)/1000.0;
   
   				//*********************************
   				150: // kl
   				//*********************************
   					iTotalizerPresetValueTemp := iTotalizerPresetValue;
   
   				else // Base unit
   					iTotalizerPresetValueTemp := iTotalizerPresetValue;
   
   			end_case;
   
   
   		 	COP(iTotalizerPresetValueTemp,SimulationDINT,1);
   
   			DataToSend[6].0 :=  SimulationDINT.24;
   			DataToSend[6].1 :=  SimulationDINT.25;
   			DataToSend[6].2 :=  SimulationDINT.26;
   			DataToSend[6].3 :=  SimulationDINT.27;
   			DataToSend[6].4 :=  SimulationDINT.28;
   			DataToSend[6].5 :=  SimulationDINT.29;
   			DataToSend[6].6 :=  SimulationDINT.30;
   			DataToSend[6].7 :=  SimulationDINT.31;
   			DataToSend[6].8 :=  SimulationDINT.16;
   			DataToSend[6].9 :=  SimulationDINT.17;
   			DataToSend[6].10 := SimulationDINT.18;
   			DataToSend[6].11 := SimulationDINT.19;
   			DataToSend[6].12 := SimulationDINT.20;
   			DataToSend[6].13 := SimulationDINT.21;
   			DataToSend[6].14 := SimulationDINT.22;
   			DataToSend[6].15 := SimulationDINT.23;
   			DataToSend[7].0  := SimulationDINT.8;
   			DataToSend[7].1  := SimulationDINT.9;
   			DataToSend[7].2  := SimulationDINT.10;
   			DataToSend[7].3  := SimulationDINT.11;
   			DataToSend[7].4  := SimulationDINT.12;
   			DataToSend[7].5  := SimulationDINT.13;
   			DataToSend[7].6  := SimulationDINT.14;
   			DataToSend[7].7  := SimulationDINT.15;
   			DataToSend[7].8  := SimulationDINT.0;
   			DataToSend[7].9  := SimulationDINT.1;
   			DataToSend[7].10 := SimulationDINT.2;
   			DataToSend[7].11 := SimulationDINT.3;
   			DataToSend[7].12 := SimulationDINT.4;
   			DataToSend[7].13 := SimulationDINT.5;
   			DataToSend[7].14 := SimulationDINT.6;
   			DataToSend[7].15 := SimulationDINT.7;
   
   			Trigger := TRUE;
   
   			if DeviceData.NewState then
   
   				DeviceData.StateDone := TRUE;
   
   			end_if;
   
   			if  DeviceData.CommSuccess and DeviceData.ReplayIndex = CMD_Index then
   
   				Trigger := FALSE;
   				DeviceData.OldState := DeviceData.State;
   				DeviceData.State := DeviceData.MaxState;
   				DeviceData.CommSuccess := FALSE;
   				DeviceData.AcyclicData[0] := 0;
   				DeviceData.NewState := TRUE;
   
   			 elsif DeviceData.CommTimeOut then
   
   				Temp_DINT := DeviceData.State;
   				DTOS(Temp_DINT, temp_string2);
   				CONCAT(temp_string1, temp_string2, qAOI_Diagnostic_String);
   
   				DeviceData.OldState := DeviceData.State;
   				DeviceData.State := DeviceData.MaxState;	//Check State
   				DeviceData.CommTimeOut := FALSE;
   				DeviceData.AcyclicData[0] := 0;
   				DeviceData.NewState := TRUE;
   
   			end_if;
   
   
   		//*********************************
   		21: // Reset totalizer
   		//*********************************
   			CMD_Index := 8281;
   			CMD_Subindex := 0;
   			CMD_Wr := TRUE;
   			CMD_Rd := FALSE;
   			CMD_ByteLength := 2;
   			DataToSend[6]:= 0;
   			DataToSend[7]:= 0;
   
   			DataToSend[6].8:= 1; // Reset
   
   			Trigger := TRUE;
   
   			if DeviceData.NewState then
   
   				DeviceData.StateDone := TRUE;
   
   			end_if;
   
   			if  DeviceData.CommSuccess and DeviceData.ReplayIndex = CMD_Index then
   
   				Trigger := FALSE;
   				DeviceData.OldState := DeviceData.State;
   				DeviceData.State := DeviceData.MaxState;
   				DeviceData.CommSuccess := FALSE;
   				DeviceData.AcyclicData[0] := 0;
   				DeviceData.NewState := TRUE;
   
   			elsif DeviceData.CommTimeOut then
   
   				Temp_DINT := DeviceData.State;
   				DTOS(Temp_DINT, temp_string2);
   				CONCAT(temp_string1, temp_string2, qAOI_Diagnostic_String);
   
   				DeviceData.OldState := DeviceData.State;
   				DeviceData.State := DeviceData.MaxState;
   				DeviceData.CommTimeOut := FALSE;
   				DeviceData.AcyclicData[0] := 0;
   				DeviceData.NewState := TRUE;
   
   			end_if;
   
   
   		//***************************************
   	    30: // Set conductivity unit
   		//***************************************
   			CMD_Index := 8298;
   			CMD_Subindex := 0;
   			CMD_Wr := TRUE;
   			CMD_Rd := FALSE;
   			CMD_ByteLength := 2;
   			DataToSend[6]:= 0;
   			DataToSend[7]:= 0;
   
   			if iUnitConductivity = 3 or iUnitConductivity = 6 or iUnitConductivity = 8 then
   
   				DataToSend[6].8 := iUnitConductivity.0;
   				DataToSend[6].9 := iUnitConductivity.1;
   				DataToSend[6].10 := iUnitConductivity.2;
   				DataToSend[6].11 := iUnitConductivity.3;
   				DataToSend[6].12 := iUnitConductivity.4;
   				DataToSend[6].13 := iUnitConductivity.5;
   				DataToSend[6].14 := iUnitConductivity.6;
   				DataToSend[6].15 := iUnitConductivity.7;
   
   				Trigger := TRUE;
   
   				if DeviceData.NewState then
   
   					DeviceData.StateDone := TRUE;
   
   				end_if;
   
   				if  DeviceData.CommSuccess and DeviceData.ReplayIndex = CMD_Index then
   
   					Trigger := FALSE;
   					DeviceData.OldState := DeviceData.State;
   					DeviceData.State := DeviceData.State + 1;	//Check State
   					DeviceData.CommSuccess := FALSE;
   					DeviceData.AcyclicData[0] := 0;
   					DeviceData.NewState := TRUE;
   
   			 	elsif DeviceData.CommTimeOut then
   
   					Temp_DINT := DeviceData.State;
   					DTOS(Temp_DINT, temp_string2);
   					CONCAT(temp_string1, temp_string2, qAOI_Diagnostic_String);
   
   					DeviceData.OldState := DeviceData.State;
   					DeviceData.State := DeviceData.State + 1;	//Check State
   					DeviceData.CommTimeOut := FALSE;
   					DeviceData.AcyclicData[0] := 0;
   					DeviceData.NewState := TRUE;
   
   				end_if;
   
   			else
   
   					Temp_DINT := DeviceData.State;
   					DTOS(Temp_DINT, temp_string2);
   					CONCAT(temp_string1, temp_string2, qAOI_Diagnostic_String);
   
   					DeviceData.OldState := DeviceData.State;
   					DeviceData.State := DeviceData.State + 1;
   					DeviceData.CommTimeOut := FALSE;
   					DeviceData.AcyclicData[0] := 0;
   					DeviceData.NewState := TRUE;
   
   	        end_if;
   
   
   		//***************************************
   	    31: // Set totalizer unit
   		//***************************************
   			CMD_Index := 8282;
   			CMD_Subindex := 0;
   			CMD_Wr := TRUE;
   			CMD_Rd := FALSE;
   			CMD_ByteLength := 2;
   			DataToSend[6]:= 0;
   			DataToSend[7]:= 0;
   
   			if iUnitTotalizer = 2 or iUnitTotalizer = 4 or iUnitTotalizer = 10 or iUnitTotalizer = 11 or iUnitTotalizer = 22 or iUnitTotalizer = 150 then
   
   			 	COP(iUnitTotalizer,SimulationDINT,1);
   
   				DataToSend[6].0 :=  SimulationDINT.8;
   				DataToSend[6].1 :=  SimulationDINT.9;
   				DataToSend[6].2 :=  SimulationDINT.10;
   				DataToSend[6].3 :=  SimulationDINT.11;
   				DataToSend[6].4 :=  SimulationDINT.12;
   				DataToSend[6].5 :=  SimulationDINT.13;
   				DataToSend[6].6 :=  SimulationDINT.14;
   				DataToSend[6].7 :=  SimulationDINT.15;
   				DataToSend[6].8 :=  SimulationDINT.0;
   				DataToSend[6].9 :=  SimulationDINT.1;
   				DataToSend[6].10 := SimulationDINT.2;
   				DataToSend[6].11 := SimulationDINT.3;
   				DataToSend[6].12 := SimulationDINT.4;
   				DataToSend[6].13 := SimulationDINT.5;
   				DataToSend[6].14 := SimulationDINT.6;
   				DataToSend[6].15 := SimulationDINT.7;
   
   				Trigger := TRUE;
   
   				if DeviceData.NewState then
   
   					DeviceData.StateDone := TRUE;
   
   				end_if;
   
   				if  DeviceData.CommSuccess and DeviceData.ReplayIndex = CMD_Index then
   
   					Trigger := FALSE;
   					DeviceData.OldState := DeviceData.State;
   					DeviceData.State := DeviceData.State + 1;
   					DeviceData.CommSuccess := FALSE;
   					DeviceData.AcyclicData[0] := 0;
   					DeviceData.NewState := TRUE;
   
   			 	elsif DeviceData.CommTimeOut then
   
   					Temp_DINT := DeviceData.State;
   					DTOS(Temp_DINT, temp_string2);
   					CONCAT(temp_string1, temp_string2, qAOI_Diagnostic_String);
   
   					DeviceData.OldState := DeviceData.State;
   					DeviceData.State := DeviceData.MaxState;	//Check State
   					DeviceData.CommTimeOut := FALSE;
   					DeviceData.AcyclicData[0] := 0;
   					DeviceData.NewState := TRUE;
   
   				end_if;
   
   			else
   
   					Temp_DINT := DeviceData.State;
   					DTOS(Temp_DINT, temp_string2);
   					CONCAT(temp_string1, temp_string2, qAOI_Diagnostic_String);
   
   					DeviceData.OldState := DeviceData.State;
   					DeviceData.State := DeviceData.State + 1;
   					DeviceData.CommTimeOut := FALSE;
   					DeviceData.AcyclicData[0] := 0;
   					DeviceData.NewState := TRUE;
   
   	        end_if;
   
   
   		//***************************************
   	    32: // Set temperature unit
   		//***************************************
   			CMD_Index := 8294;
   			CMD_Subindex := 0;
   			CMD_Wr := TRUE;
   			CMD_Rd := FALSE;
   			CMD_ByteLength := 2;
   			DataToSend[6]:= 0;
   			DataToSend[7]:= 0;
   
   			if iUnitTemperature = 32 or iUnitTemperature = 33 then
   
   				DataToSend[6].8 := iUnitTemperature.0;
   				DataToSend[6].9 := iUnitTemperature.1;
   				DataToSend[6].10 := iUnitTemperature.2;
   				DataToSend[6].11 := iUnitTemperature.3;
   				DataToSend[6].12 := iUnitTemperature.4;
   				DataToSend[6].13 := iUnitTemperature.5;
   				DataToSend[6].14 := iUnitTemperature.6;
   				DataToSend[6].15 := iUnitTemperature.7;
   
   				Trigger := TRUE;
   
   				if DeviceData.NewState then
   
   					DeviceData.StateDone := TRUE;
   
   				end_if;
   
   				if  DeviceData.CommSuccess and DeviceData.ReplayIndex = CMD_Index then
   
   					Trigger := FALSE;
   					DeviceData.OldState := DeviceData.State;
   					DeviceData.State := DeviceData.State + 1;
   					DeviceData.CommSuccess := FALSE;
   					DeviceData.AcyclicData[0] := 0;
   					DeviceData.NewState := TRUE;
   
   			 	elsif DeviceData.CommTimeOut then
   
   					Temp_DINT := DeviceData.State;
   					DTOS(Temp_DINT, temp_string2);
   					CONCAT(temp_string1, temp_string2, qAOI_Diagnostic_String);
   
   					DeviceData.OldState := DeviceData.State;
   					DeviceData.State := DeviceData.MaxState;	//Check State
   					DeviceData.CommTimeOut := FALSE;
   					DeviceData.AcyclicData[0] := 0;
   					DeviceData.NewState := TRUE;
   
   				end_if;
   
   			else
   
   					Temp_DINT := DeviceData.State;
   					DTOS(Temp_DINT, temp_string2);
   					CONCAT(temp_string1, temp_string2, qAOI_Diagnostic_String);
   
   					DeviceData.OldState := DeviceData.State;
   					DeviceData.State := DeviceData.State + 1;
   					DeviceData.CommTimeOut := FALSE;
   					DeviceData.AcyclicData[0] := 0;
   					DeviceData.NewState := TRUE;
   
   	        end_if;
   
   
   		//***************************************
   	    33: // Set flow velocity unit
   		//***************************************
   			CMD_Index := 8297;
   			CMD_Subindex := 0;
   			CMD_Wr := TRUE;
   			CMD_Rd := FALSE;
   			CMD_ByteLength := 2;
   			DataToSend[6]:= 0;
   			DataToSend[7]:= 0;
   
   			// Split test in 2 due to too many "or" operators use (Limited to 6 "or")
   			if iUnitFlowVelocity = 21 or iUnitFlowVelocity = 22 or iUnitFlowVelocity = 50
   				or iUnitFlowVelocity = 114 or iUnitFlowVelocity = 115 or iUnitFlowVelocity = 116 or iUnitFlowVelocity = 120 then
   
   				unit_check := TRUE;
   
   			elsif iUnitFlowVelocity = 240 then
   
   				unit_check := TRUE;
   
   			else
   
   				unit_check := FALSE;
   
   			end_if;
   
   			if unit_check then
   
   			 	COP(iUnitFlowVelocity,SimulationDINT,1);
   
   				DataToSend[6].0 :=  SimulationDINT.8;
   				DataToSend[6].1 :=  SimulationDINT.9;
   				DataToSend[6].2 :=  SimulationDINT.10;
   				DataToSend[6].3 :=  SimulationDINT.11;
   				DataToSend[6].4 :=  SimulationDINT.12;
   				DataToSend[6].5 :=  SimulationDINT.13;
   				DataToSend[6].6 :=  SimulationDINT.14;
   				DataToSend[6].7 :=  SimulationDINT.15;
   				DataToSend[6].8 :=  SimulationDINT.0;
   				DataToSend[6].9 :=  SimulationDINT.1;
   				DataToSend[6].10 := SimulationDINT.2;
   				DataToSend[6].11 := SimulationDINT.3;
   				DataToSend[6].12 := SimulationDINT.4;
   				DataToSend[6].13 := SimulationDINT.5;
   				DataToSend[6].14 := SimulationDINT.6;
   				DataToSend[6].15 := SimulationDINT.7;
   
   				Trigger := TRUE;
   
   				if DeviceData.NewState then
   
   					DeviceData.StateDone := TRUE;
   
   				end_if;
   
   				if  DeviceData.CommSuccess and DeviceData.ReplayIndex = CMD_Index then
   
   					Trigger := FALSE;
   					DeviceData.OldState := DeviceData.State;
   					DeviceData.State := DeviceData.State + 1;
   					DeviceData.CommSuccess := FALSE;
   					DeviceData.AcyclicData[0] := 0;
   					DeviceData.NewState := TRUE;
   
   			 	elsif DeviceData.CommTimeOut then
   
   					Temp_DINT := DeviceData.State;
   					DTOS(Temp_DINT, temp_string2);
   					CONCAT(temp_string1, temp_string2, qAOI_Diagnostic_String);
   
   					DeviceData.OldState := DeviceData.State;
   					DeviceData.State := DeviceData.MaxState;	//Check State
   					DeviceData.CommTimeOut := FALSE;
   					DeviceData.AcyclicData[0] := 0;
   					DeviceData.NewState := TRUE;
   
   				end_if;
   
   			else
   
   					Temp_DINT := DeviceData.State;
   					DTOS(Temp_DINT, temp_string2);
   					CONCAT(temp_string1, temp_string2, qAOI_Diagnostic_String);
   
   					DeviceData.OldState := DeviceData.State;
   					DeviceData.State := DeviceData.State + 1;
   					DeviceData.CommTimeOut := FALSE;
   					DeviceData.AcyclicData[0] := 0;
   					DeviceData.NewState := TRUE;
   
   	        end_if;
   
   		//***************************************
   	    34: // Set volume flow unit
   		//***************************************
   			CMD_Index := 8295;
   			CMD_Subindex := 0;
   			CMD_Wr := TRUE;
   			CMD_Rd := FALSE;
   			CMD_ByteLength := 2;
   			DataToSend[6]:= 0;
   			DataToSend[7]:= 0;
   
   			if iUnitVolumeFlow = 16 or iUnitVolumeFlow = 17 or iUnitVolumeFlow = 18
   				or iUnitVolumeFlow = 19 or iUnitVolumeFlow = 24 or iUnitVolumeFlow = 41 then
   
   				DataToSend[6].8 := iUnitVolumeFlow.0;
   				DataToSend[6].9 := iUnitVolumeFlow.1;
   				DataToSend[6].10 := iUnitVolumeFlow.2;
   				DataToSend[6].11 := iUnitVolumeFlow.3;
   				DataToSend[6].12 := iUnitVolumeFlow.4;
   				DataToSend[6].13 := iUnitVolumeFlow.5;
   				DataToSend[6].14 := iUnitVolumeFlow.6;
   				DataToSend[6].15 := iUnitVolumeFlow.7;
   
   				Trigger := TRUE;
   
   				if DeviceData.NewState then
   
   					DeviceData.StateDone := TRUE;
   
   				end_if;
   
   				if  DeviceData.CommSuccess and DeviceData.ReplayIndex = CMD_Index then
   
   					Trigger := FALSE;
   					DeviceData.OldState := DeviceData.State;
   					DeviceData.State := DeviceData.State + 1;
   					DeviceData.CommSuccess := FALSE;
   					DeviceData.AcyclicData[0] := 0;
   					DeviceData.NewState := TRUE;
   
   			 	elsif DeviceData.CommTimeOut then
   
   					Temp_DINT := DeviceData.State;
   					DTOS(Temp_DINT, temp_string2);
   					CONCAT(temp_string1, temp_string2, qAOI_Diagnostic_String);
   
   					DeviceData.OldState := DeviceData.State;
   					DeviceData.State := DeviceData.MaxState;	//Check State
   					DeviceData.CommTimeOut := FALSE;
   					DeviceData.AcyclicData[0] := 0;
   					DeviceData.NewState := TRUE;
   
   				end_if;
   
   			else
   
   					Temp_DINT := DeviceData.State;
   					DTOS(Temp_DINT, temp_string2);
   					CONCAT(temp_string1, temp_string2, qAOI_Diagnostic_String);
   
   					DeviceData.OldState := DeviceData.State;
   					DeviceData.State := DeviceData.State + 1;
   					DeviceData.CommTimeOut := FALSE;
   					DeviceData.AcyclicData[0] := 0;
   					DeviceData.NewState := TRUE;
   
   	        end_if;
   
   
   		//***************************************
   	    35: // Read conductivity unit
   		//***************************************
   			CMD_Index := 8298;
   			CMD_Subindex := 0;
   			CMD_Wr := FALSE;
   			CMD_Rd := TRUE;
   			CMD_ByteLength := 2;
   			Trigger := TRUE;
   
   			if DeviceData.NewState then
   
   				DeviceData.StateDone := TRUE;
   
   			end_if;
   
   			if  DeviceData.CommSuccess and DeviceData.ReplayIndex = CMD_Index then
   
   				qUnitConductivity.0	:= DeviceData.AcyclicData[0].0;
   				qUnitConductivity.1	:= DeviceData.AcyclicData[0].1;
   				qUnitConductivity.2	:= DeviceData.AcyclicData[0].2;
   				qUnitConductivity.3	:= DeviceData.AcyclicData[0].3;
   				qUnitConductivity.4	:= DeviceData.AcyclicData[0].4;
   				qUnitConductivity.5	:= DeviceData.AcyclicData[0].5;
   				qUnitConductivity.6	:= DeviceData.AcyclicData[0].6;
   				qUnitConductivity.7	:= DeviceData.AcyclicData[0].7;
   
   				Trigger := FALSE;
   				DeviceData.OldState := DeviceData.State;
   				DeviceData.State := DeviceData.State + 1;
   				DeviceData.CommSuccess := FALSE;
   				DeviceData.AcyclicData[0] := 0;
   				DeviceData.NewState := TRUE;
   
   			 elsif DeviceData.CommTimeOut then
   
   				Temp_DINT := DeviceData.State;
   				DTOS(Temp_DINT, temp_string2);
   				CONCAT(temp_string1, temp_string2, qAOI_Diagnostic_String);
   
   				DeviceData.OldState := DeviceData.State;
   				DeviceData.State := DeviceData.MaxState;
   				DeviceData.CommTimeOut := FALSE;
   				DeviceData.AcyclicData[0] := 0;
   				DeviceData.NewState := TRUE;
   
   			end_if;
   
   
   		//***************************************
   	    36: // Read totalizer unit
   		//***************************************
   			CMD_Index := 8282;
   			CMD_Subindex := 0;
   			CMD_Wr := FALSE;
   			CMD_Rd := TRUE;
   			CMD_ByteLength := 2;
   			Trigger := TRUE;
   
   			if DeviceData.NewState then
   
   				DeviceData.StateDone := TRUE;
   
   			end_if;
   
   			if  DeviceData.CommSuccess and DeviceData.ReplayIndex = CMD_Index then
   
   				COP(DeviceData.AcyclicData[0], qUnitTotalizer, 1);
   
   				Trigger := FALSE;
   				DeviceData.OldState := DeviceData.State;
   				DeviceData.State := DeviceData.State + 1;
   				DeviceData.CommSuccess := FALSE;
   				DeviceData.AcyclicData[0] := 0;
   				DeviceData.NewState := TRUE;
   
   			 elsif DeviceData.CommTimeOut then
   
   				Temp_DINT := DeviceData.State;
   				DTOS(Temp_DINT, temp_string2);
   				CONCAT(temp_string1, temp_string2, qAOI_Diagnostic_String);
   
   				DeviceData.OldState := DeviceData.State;
   				DeviceData.State := DeviceData.MaxState;
   				DeviceData.CommTimeOut := FALSE;
   				DeviceData.AcyclicData[0] := 0;
   				DeviceData.NewState := TRUE;
   
   			end_if;
   
   
   		//***************************************
   	    37: // Read temperature unit
   		//***************************************
   			CMD_Index := 8294;
   			CMD_Subindex := 0;
   			CMD_Wr := FALSE;
   			CMD_Rd := TRUE;
   			CMD_ByteLength := 2;
   			Trigger := TRUE;
   
   			if DeviceData.NewState then
   
   				DeviceData.StateDone := TRUE;
   
   			end_if;
   
   			if  DeviceData.CommSuccess and DeviceData.ReplayIndex = CMD_Index then
   
   				qUnitTemperature.0	:= DeviceData.AcyclicData[0].0;
   				qUnitTemperature.1	:= DeviceData.AcyclicData[0].1;
   				qUnitTemperature.2	:= DeviceData.AcyclicData[0].2;
   				qUnitTemperature.3	:= DeviceData.AcyclicData[0].3;
   				qUnitTemperature.4	:= DeviceData.AcyclicData[0].4;
   				qUnitTemperature.5	:= DeviceData.AcyclicData[0].5;
   				qUnitTemperature.6	:= DeviceData.AcyclicData[0].6;
   				qUnitTemperature.7	:= DeviceData.AcyclicData[0].7;
   
   				Trigger := FALSE;
   				DeviceData.OldState := DeviceData.State;
   				DeviceData.State := DeviceData.State + 1;
   				DeviceData.CommSuccess := FALSE;
   				DeviceData.AcyclicData[0] := 0;
   				DeviceData.NewState := TRUE;
   
   			 elsif DeviceData.CommTimeOut then
   
   				Temp_DINT := DeviceData.State;
   				DTOS(Temp_DINT, temp_string2);
   				CONCAT(temp_string1, temp_string2, qAOI_Diagnostic_String);
   
   				DeviceData.OldState := DeviceData.State;
   				DeviceData.State := DeviceData.MaxState;
   				DeviceData.CommTimeOut := FALSE;
   				DeviceData.AcyclicData[0] := 0;
   				DeviceData.NewState := TRUE;
   
   			end_if;
   
   
   		//***************************************
   	    38: // Read flow velocity unit
   		//***************************************
   			CMD_Index := 8297;
   			CMD_Subindex := 0;
   			CMD_Wr := FALSE;
   			CMD_Rd := TRUE;
   			CMD_ByteLength := 2;
   			Trigger := TRUE;
   
   			if DeviceData.NewState then
   
   				DeviceData.StateDone := TRUE;
   
   			end_if;
   
   			if  DeviceData.CommSuccess and DeviceData.ReplayIndex = CMD_Index then
   
   				COP(DeviceData.AcyclicData[0], qUnitFlowVelocity, 1);
   
   				Trigger := FALSE;
   				DeviceData.OldState := DeviceData.State;
   				DeviceData.State := DeviceData.State + 1;
   				DeviceData.CommSuccess := FALSE;
   				DeviceData.AcyclicData[0] := 0;
   				DeviceData.NewState := TRUE;
   
   			 elsif DeviceData.CommTimeOut then
   
   				Temp_DINT := DeviceData.State;
   				DTOS(Temp_DINT, temp_string2);
   				CONCAT(temp_string1, temp_string2, qAOI_Diagnostic_String);
   
   				DeviceData.OldState := DeviceData.State;
   				DeviceData.State := DeviceData.MaxState;
   				DeviceData.CommTimeOut := FALSE;
   				DeviceData.AcyclicData[0] := 0;
   				DeviceData.NewState := TRUE;
   
   			end_if;
   
   
   		//***************************************
   	    39: // Read volume flow unit
   		//***************************************
   			CMD_Index := 8295;
   			CMD_Subindex := 0;
   			CMD_Wr := FALSE;
   			CMD_Rd := TRUE;
   			CMD_ByteLength := 2;
   			Trigger := TRUE;
   
   			if DeviceData.NewState then
   
   				DeviceData.StateDone := TRUE;
   
   			end_if;
   
   			if  DeviceData.CommSuccess and DeviceData.ReplayIndex = CMD_Index then
   
   				qUnitVolumeFlow.0	:= DeviceData.AcyclicData[0].0;
   				qUnitVolumeFlow.1	:= DeviceData.AcyclicData[0].1;
   				qUnitVolumeFlow.2	:= DeviceData.AcyclicData[0].2;
   				qUnitVolumeFlow.3	:= DeviceData.AcyclicData[0].3;
   				qUnitVolumeFlow.4	:= DeviceData.AcyclicData[0].4;
   				qUnitVolumeFlow.5	:= DeviceData.AcyclicData[0].5;
   				qUnitVolumeFlow.6	:= DeviceData.AcyclicData[0].6;
   				qUnitVolumeFlow.7	:= DeviceData.AcyclicData[0].7;
   
   				Trigger := FALSE;
   				DeviceData.OldState := DeviceData.State;
   				DeviceData.State := DeviceData.MaxState;
   				DeviceData.CommSuccess := FALSE;
   				DeviceData.AcyclicData[0] := 0;
   				DeviceData.NewState := TRUE;
   
   				if not init_qUnits then
   
   					init_qUnits := TRUE;
   					DeviceData.State := 90;
   
   				end_if;
   
   			 elsif DeviceData.CommTimeOut then
   
   				Temp_DINT := DeviceData.State;
   				DTOS(Temp_DINT, temp_string2);
   				CONCAT(temp_string1, temp_string2, qAOI_Diagnostic_String);
   
   				DeviceData.OldState := DeviceData.State;
   				DeviceData.State := DeviceData.MaxState;
   				DeviceData.CommTimeOut := FALSE;
   				DeviceData.AcyclicData[0] := 0;
   				DeviceData.NewState := TRUE;
   
   			end_if;
   
   
   		//*********************************
   		90: // Active diagnostic
   		//*********************************
   
   			CMD_Index := 8304;
   			CMD_Subindex := 0;
   			CMD_Wr := FALSE;
   			CMD_Rd := TRUE;
   			CMD_ByteLength := 4;
   			DataToSend[6]:= 0;
   			DataToSend[7]:= 0;
   			Trigger := TRUE;
   
   			if DeviceData.NewState then
   				DeviceData.StateDone := TRUE;
   			end_if;
   
   			if  DeviceData.CommSuccess and DeviceData.ReplayIndex = CMD_Index then
   
   				qActual_Diagnostics_Code	:= DeviceData.AcyclicData[0];
   
   				case qActual_Diagnostics_Code of
   				 	0:
   			            qActual_Diagnostics_String := '--------';
   			        16777217:
   			            qActual_Diagnostics_String := 'F453 Flow override active';
   			        16777219:
   			            qActual_Diagnostics_String := 'F411 Up-/download active';
   			        16777429:
   			            qActual_Diagnostics_String := 'F180 Temperature sensor defective';
   			        16777500:
   			            qActual_Diagnostics_String := 'F181 Sensor connection faulty';
   			        16777547:
   			            qActual_Diagnostics_String := 'F201 Electronics faulty';
   			        16777583:
   			            qActual_Diagnostics_String := 'F283 Memory content inconsistent';
   			        25165825:
   			            qActual_Diagnostics_String := 'F453 Flow override active';
   			        25165827:
   			            qActual_Diagnostics_String := 'F411 Up-/download active';
   			        25166037:
   			            qActual_Diagnostics_String := 'F180 Temperature sensor defective';
   			        25166108:
   			            qActual_Diagnostics_String := 'F181 Sensor connection faulty';
   			        25166155:
   			            qActual_Diagnostics_String := 'F201 Electronics faulty';
   			        25166191:
   			            qActual_Diagnostics_String := 'F283 Memory content inconsistent';
   			        33554579:
   			            qActual_Diagnostics_String := 'C485 Process variable simulation active';
   			        41943187:
   			            qActual_Diagnostics_String := 'C485 Process variable simulation active';
   			        134217812:
   			            qActual_Diagnostics_String := 'S841 Operating range';
   			        134217868:
   			            qActual_Diagnostics_String := 'S443 Pulse output saturated';
   			        134217874:
   			            qActual_Diagnostics_String := 'S962 Pipe empty';
   			        134217881:
   			            qActual_Diagnostics_String := 'S441 Current output saturated';
   			        134217925:
   			            qActual_Diagnostics_String := 'S834 Process temperature too high';
   			        134217926:
   			            qActual_Diagnostics_String := 'S835 Process temperature too low';
   			        134219072:
   			            qActual_Diagnostics_String := 'S880 Output overloaded';
   			        142606420:
   			            qActual_Diagnostics_String := 'S841 Operating range';
   			        142606476:
   			            qActual_Diagnostics_String := 'S443 Pulse output saturated';
   			        142606482:
   			            qActual_Diagnostics_String := 'S962 Pipe empty';
   			        142606489:
   			            qActual_Diagnostics_String := 'S441 Current output saturated';
   			        142606533:
   			            qActual_Diagnostics_String := 'S834 Process temperature too high';
   			        142606534:
   			            qActual_Diagnostics_String := 'S835 Process temperature too low';
   			        142607680:
   			            qActual_Diagnostics_String := 'S880 Output overloaded';
   
   				else
   
   					qActual_Diagnostics_String := 'Error Code unknown';
   
   				end_case;
   
   				Trigger := 0;
   				DeviceData.OldState := DeviceData.State;
   		        DeviceData.State := DeviceData.MaxState;
   				DeviceData.CommSuccess := FALSE;
   				DeviceData.AcyclicData[0] := 0;
   				DeviceData.NewState := TRUE;
   
   
   			 elsif DeviceData.CommTimeOut then
   
   				temp_string1 := 'Error in step ';
   				Temp_DINT := DeviceData.State;
   				DTOS(Temp_DINT, temp_string2);
   				CONCAT(temp_string1, temp_string2, qAOI_Diagnostic_String);
   
   				DeviceData.OldState := DeviceData.State;
   				DeviceData.State := DeviceData.MaxState;	//Check State
   				DeviceData.CommTimeOut := FALSE;
   				DeviceData.AcyclicData[0] := 0;
   				DeviceData.NewState := TRUE;
   
   		    end_if;
   
   
   		//*********************************
   		98: // End Step Trigger Guard
   		//*********************************
   
   				DeviceData.State := 0;
   				CommAOIBusy := 0;
   				DeviceAOISendRequest.[DeviceData.DevicePort] := FALSE;
   				ActiveComPort := 0;
   				ActiveAOI := FALSE;
   				DataToSend[0] := 0;
   				DataToSend[1] := 0;
   				DataToSend[2] := 0;
   				DataToSend[3] := 0;
   				DataToSend[4] := 0;
   				DataToSend[5] := 0;
    				DataToSend[6] := 0;
   				DataToSend[7] := 0;
    				DataToSend[8] := 0;
   				DataToSend[9] := 0;
   				DeviceData.StateDone := FALSE;
   				Skip := FALSE;
   				DeviceData.State := 0;
   				firstTimeDone := FALSE;
   				DeviceData.NewState := FALSE;
   				DeviceData.OldState := 0;
   				ActiveAOI := FALSE;
   
   				if SimActive then
   
   					SimActive := FALSE;
   					SimChanged := FALSE;
   
   				elsif TotPresetActive then
   
   					TotPresetActive := FALSE;
   					TotPresetChanged := FALSE;
   
   				elsif TotResetActive then
   
   					TotResetActive := FALSE;
   					TotResetChanged := FALSE;
   
   				elsif ReadProcessDataActive then
   
   					ReadProcessDataActive := FALSE;
   					ReadProcessDataChanged := FALSE;
   
   				elsif UnitActive then
   
   					UnitActive := FALSE;
   					UnitChanged := FALSE;
   
   				elsif CondStatusActive then
   
   					CondStatusActive := FALSE;
   					CondStatusChanged := FALSE;
   
   				end_if;
   
   	end_case;
   
   	end_if;
   
   	//*************************
   	// Execution Area
   	//*************************
   	if DeviceData.State > StateMin and DeviceData.State < DeviceData.MaxState then
   
   		DataToSend[2] := DeviceData.DevicePort;
   		DataToSend[3] := CMD_Index;
   		DataToSend[4] := CMD_Subindex;
   		DataToSend[5].0 := CMD_Rd;
   		DataToSend[5].1 := CMD_Wr;
   		DataToSend[5].8 := CMD_ByteLength.0;  // Bits for the Length of the Data
   		DataToSend[5].9 := CMD_ByteLength.1;
   		DataToSend[5].10 := CMD_ByteLength.2;
   		DataToSend[5].11 := CMD_ByteLength.3;
   		DataToSend[5].12 := CMD_ByteLength.4;
   		DataToSend[5].13 := CMD_ByteLength.5;
   		DataToSend[5].14 := CMD_ByteLength.6;
   		DataToSend[5].15 := CMD_ByteLength.7;
   		DataToSend[5].7 := Trigger;
   
   		qCommError := CommError;
   
   	end_if;
   
   
   end_if;
   
   
END_ROUTINE
END_ADD_ON_INSTRUCTION
